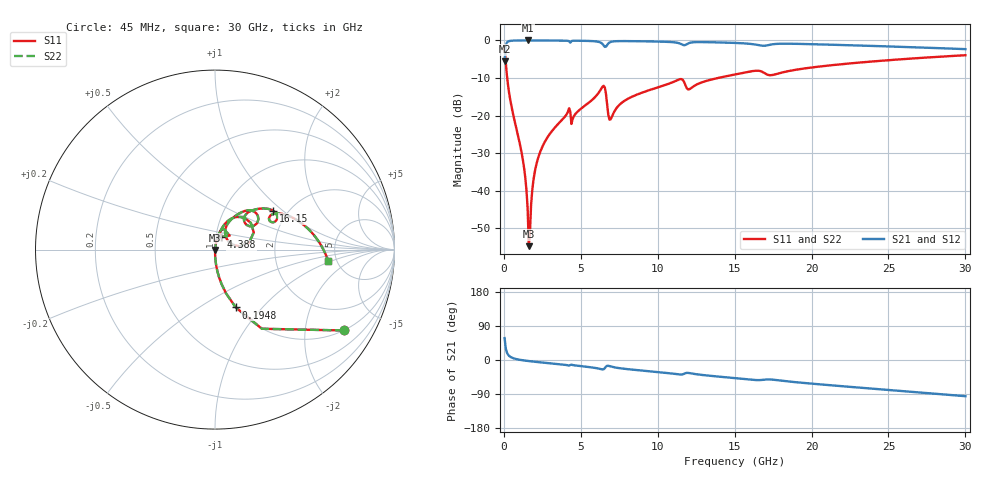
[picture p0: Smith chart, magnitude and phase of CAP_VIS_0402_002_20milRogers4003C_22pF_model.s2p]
! S-parameter model data by Modelithics Inc.  support@modelithics.com  813-866-6335  Tampa FL USA
! S-Parameter data specifications:
! Substrate: 20-mil Rogers 4003C, substrate thickness, H=0.508mm, Dielectric constant, Er=3.75
! PCB Mounting Pad Footprint: Pad width, PadW=0.50mm , Pad length, PadL=0.50mm , Pad gap, PadG (edge-to-edge)=0.40mm , Reference planes=1.4mm apart
! Created Wed Nov 18 12:52:57 2015
# hz S ma R 50
! 2 Port Network Data from SP1.SP block
! freq  magS11  angS11  magS21  angS21  magS12  angS12  magS22  angS22
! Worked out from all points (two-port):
!   401 points, 45 MHz to 30 GHz, reference 50 ohm
!   highest |S21| = -0.01 dB at 1.543 GHz (marker M1); lowest = -5.5 dB at 45 MHz (marker M2)
!   |S21| within 3 dB of the highest: 89.76 MHz to end of sweep
!   lowest |S11| = -54.8 dB at 1.618 GHz (marker M3), VSWR 1.00, Z = 50.1 - j0.15 ohm
!   |S11| at or under -10 dB: 214 MHz to 13.92 GHz (13.7 GHz wide, 194 % of centre)
!   |S22| runs from -54.8 to -1.4 dB; largest |S21 - S12| = 0
!   S11 on the Smith chart (normalised r, x): 45 MHz: 1.00, -3.19; 194.8 MHz: 1.00, -0.73; 4.388 GHz: 1.06, +0.15; 16.15 GHz: 1.68, +0.86; 30 GHz: 4.26, -0.94
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4.5e7  0.8477 -32.1  0.5303 57.9  0.5303 57.9  0.8477 -32.1
1.94775e8  0.3423 -70.3  0.9392 19.7  0.9392 19.7  0.3423 -70.3
4.194375e8  0.1584 -81.4  0.9868 8.4  0.9868 8.4  0.1584 -81.4
1.2432e9  0.02491 -88.6  0.9987 -0.8  0.9987 -0.8  0.02491 -88.6
1.54275e9  0.005727 -81.6  0.9989 -2.5  0.9989 -2.5  0.005727 -81.6
1.617638e9  0.001824 -55.3  0.9988 -2.9  0.9988 -2.9  0.001824 -55.3
1.767412e9  0.006478 76.1  0.9988 -3.6  0.9988 -3.6  0.006478 76.1
2.066962e9  0.02047 81.6  0.9985 -4.9  0.9985 -4.9  0.02047 81.6
2.4414e9  0.03615 81.3  0.9979 -6.5  0.9979 -6.5  0.03615 81.3
4.088925e9  0.1049 74.3  0.9902 -13.4  0.9902 -13.4  0.1049 74.3
4.388475e9  0.07733 64.4  0.9792 -12.3  0.9792 -12.3  0.07733 64.4
5.062462e9  0.1257 72.1  0.9886 -16.4  0.9886 -16.4  0.1257 72.1
6.410438e9  0.2421 46.2  0.8947 -24.9  0.8947 -24.9  0.2421 46.2
6.93465e9  0.08893 43.2  0.9527 -17.0  0.9527 -17.0  0.08893 43.2
7.908188e9  0.1604 63.8  0.9795 -23.6  0.9795 -23.6  0.1604 63.8
1.007992e10  0.2399 56.5  0.9649 -32.2  0.9649 -32.2  0.2399 56.5
1.210189e10  0.2268 44.2  0.9314 -34.8  0.9314 -34.8  0.2268 44.2
1.50225e10  0.3522 40.6  0.9262 -47.9  0.9262 -47.9  0.3522 40.6
1.614581e10  0.39 33.7  0.8933 -52.3  0.8933 -52.3  0.39 33.7
2.003996e10  0.437 26.4  0.8906 -62.5  0.8906 -62.5  0.437 26.4
2.505742e10  0.5465 10.1  0.831 -79.3  0.831 -79.3  0.5465 10.1
3e10  0.6352 -6.0  0.7657 -95.5  0.7657 -95.5  0.6352 -6.0
